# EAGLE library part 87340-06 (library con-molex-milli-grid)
RECEPTACAL
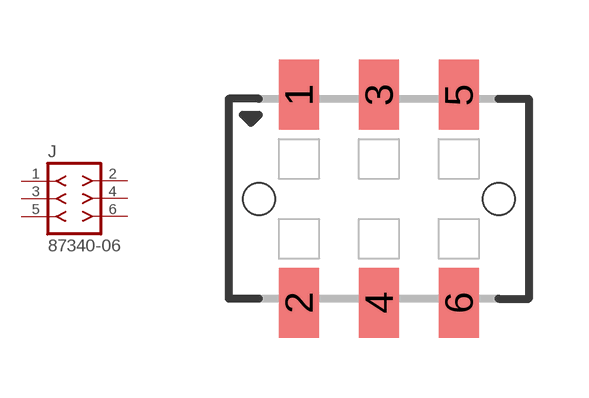
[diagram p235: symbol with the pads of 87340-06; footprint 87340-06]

Designator prefix J

## 87340-06  [87340-06]
1  1  pas
2  2  pas
3  3  pas
4  4  pas
5  5  pas
6  6  pas

## Footprint 87340-06 (pad centres in mm)
RECEPTACAL SMD Dual Row, Vertical, Low Profile
smd 1 x 1.75: 1 -2,2.6; 2 -2,-2.6; 3 0,2.6; 4 0,-2.6; 5 2,2.6; 6 2,-2.6
hole 0.8 at -3,0
hole 0.8 at 3,0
